PROGRAM P_Prog3
VAR

	fbKL6401 					: FB_LON_KL6401;

	fbREAD_063		: FB_READ_063_SNVT_temp_f;
	fbSEND_063		: FB_SEND_063_SNVT_temp_f;

	fbREAD_064		: FB_READ_064_SNVT_time_f;
	fbSEND_064		: FB_SEND_064_SNVT_time_f;

	fbREAD_065		: FB_READ_065_SNVT_vol_f;
	fbSEND_065		: FB_SEND_065_SNVT_vol_f;

	fbREAD_066		: FB_READ_066_SNVT_volt_f;
	fbSEND_066		: FB_SEND_066_SNVT_volt_f;

	fbREAD_067		: FB_READ_067_SNVT_btu_f;
	fbSEND_067		: FB_SEND_067_SNVT_btu_f;

	fbREAD_068		: FB_READ_068_SNVT_elec_whr_f;
	fbSEND_068		: FB_SEND_068_SNVT_elec_whr_f;

	fbREAD_069		: FB_READ_069_SNVT_config_src;
	fbSEND_069		: FB_SEND_069_SNVT_config_src;

	fbREAD_070		: FB_READ_070_SNVT_color;
	fbSEND_070		: FB_SEND_070_SNVT_color;

	fbREAD_071		: FB_READ_071_SNVT_grammage;
	fbSEND_071		: FB_SEND_071_SNVT_grammage;

	fbREAD_072		: FB_READ_072_SNVT_grammage_f;
	fbSEND_072		: FB_SEND_072_SNVT_grammage_f;

	fbREAD_073		: FB_READ_073_SNVT_file_req;
	fbSEND_073		: FB_SEND_073_SNVT_file_req;

	fbREAD_074		: FB_READ_074_SNVT_file_status;
	fbSEND_074		: FB_SEND_074_SNVT_file_status;

	fbREAD_075		: FB_READ_075_SNVT_freq_f;
	fbSEND_075		: FB_SEND_075_SNVT_freq_f;

	fbREAD_076		: FB_READ_076_SNVT_freq_hz;
	fbSEND_076		: FB_SEND_076_SNVT_freq_hz;

	fbREAD_077		: FB_READ_077_SNVT_freq_kilohz;
	fbSEND_077		: FB_SEND_077_SNVT_freq_kilohz;

	fbREAD_078		: FB_READ_078_SNVT_freq_milhz;
	fbSEND_078		: FB_SEND_078_SNVT_freq_milhz;

	fbREAD_079		: FB_READ_079_SNVT_lux;
	fbSEND_079		: FB_SEND_079_SNVT_lux;
(*
	fbREAD_080		: FB_READ_080;
	fbSEND_080		: FB_SEND_080_SNVT_angle_vel_f;
*)
	fbREAD_081		: FB_READ_081_SNVT_lev_percent;
	fbSEND_081		: FB_SEND_081_SNVT_lev_percent;

	fbREAD_082		: FB_READ_082_SNVT_multiplier;
	fbSEND_082		: FB_SEND_082_SNVT_multiplier;

	fbREAD_083		: FB_READ_083_SNVT_state;
	fbSEND_083		: FB_SEND_083_SNVT_state;

	fbREAD_084		: FB_READ_084_SNVT_time_stamp;
	fbSEND_084		: FB_SEND_084_SNVT_time_stamp;

	fbREAD_085		: FB_READ_085_SNVT_zerospan;
	fbSEND_085		: FB_SEND_085_SNVT_zerospan;

	fbREAD_086		: FB_READ_086_SNVT_magcard;
	fbSEND_086		: FB_SEND_086_SNVT_magcard;

	fbREAD_087		: FB_READ_087_SNVT_elapsed_tm;
	fbSEND_087		: FB_SEND_087_SNVT_elapsed_tm;

	fbREAD_088		: FB_READ_088_SNVT_alarm;
	fbSEND_088		: FB_SEND_088_SNVT_alarm;

	fbREAD_089		: FB_READ_089_SNVT_currency;
	fbSEND_089		: FB_SEND_089_SNVT_currency;

	fbREAD_090		: FB_READ_090_SNVT_file_pos;
	fbSEND_090		: FB_SEND_090_SNVT_file_pos;

	fbREAD_091		: FB_READ_091_SNVT_muldiv;
	fbSEND_091		: FB_SEND_091_SNVT_muldiv;

	fbREAD_092		: FB_READ_092_SNVT_obj_request;
	fbSEND_092		: FB_SEND_092_SNVT_obj_request;

	fbREAD_093		: FB_READ_093_SNVT_obj_status;
	fbSEND_093		: FB_SEND_093_SNVT_obj_status;

END_VAR

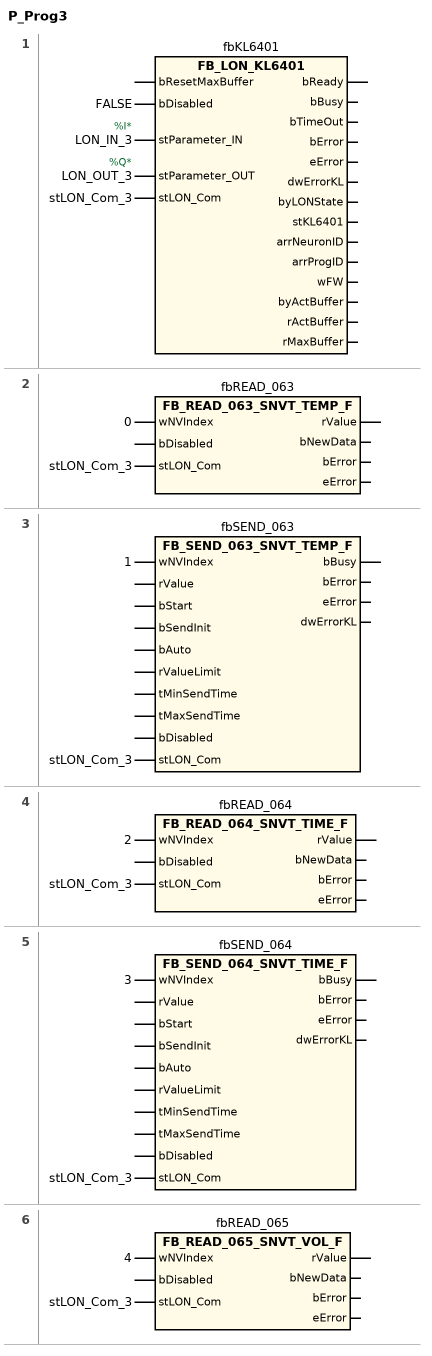
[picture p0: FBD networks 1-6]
// NETWORK 1
//   LON_IN_3: AT %I*
//   LON_OUT_3: AT %Q*
fbKL6401(
    bDisabled := FALSE,
    stParameter_IN := LON_IN_3,
    stParameter_OUT := LON_OUT_3,
    stLON_Com := stLON_Com_3); // FB_LON_KL6401

// NETWORK 2
fbREAD_063(wNVIndex := 0, stLON_Com := stLON_Com_3); // FB_READ_063_SNVT_TEMP_F

// NETWORK 3
fbSEND_063(wNVIndex := 1, stLON_Com := stLON_Com_3); // FB_SEND_063_SNVT_TEMP_F

// NETWORK 4
fbREAD_064(wNVIndex := 2, stLON_Com := stLON_Com_3); // FB_READ_064_SNVT_TIME_F

// NETWORK 5
fbSEND_064(wNVIndex := 3, stLON_Com := stLON_Com_3); // FB_SEND_064_SNVT_TIME_F

// NETWORK 6
fbREAD_065(wNVIndex := 4, stLON_Com := stLON_Com_3); // FB_READ_065_SNVT_VOL_F

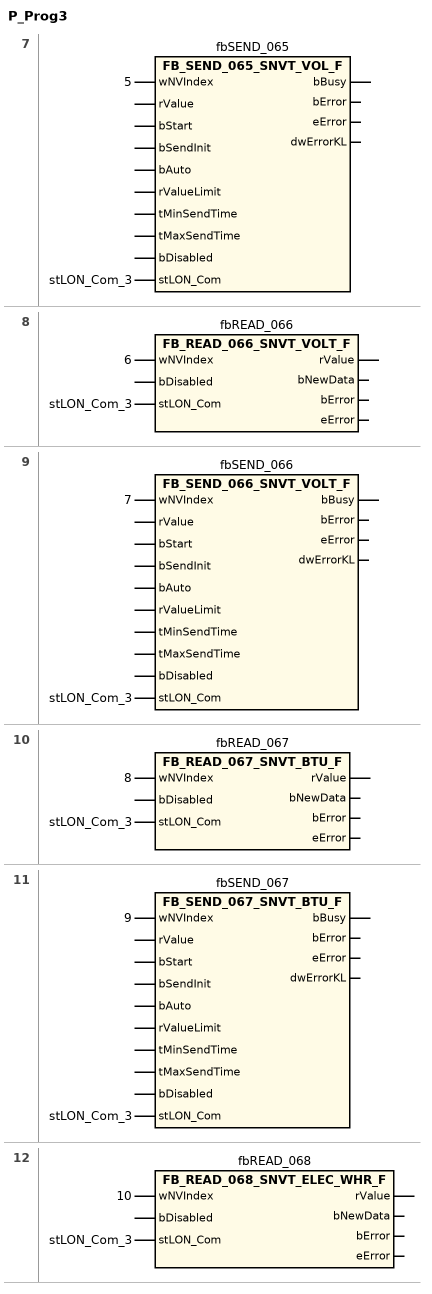
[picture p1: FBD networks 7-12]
// NETWORK 7
fbSEND_065(wNVIndex := 5, stLON_Com := stLON_Com_3); // FB_SEND_065_SNVT_VOL_F

// NETWORK 8
fbREAD_066(wNVIndex := 6, stLON_Com := stLON_Com_3); // FB_READ_066_SNVT_VOLT_F

// NETWORK 9
fbSEND_066(wNVIndex := 7, stLON_Com := stLON_Com_3); // FB_SEND_066_SNVT_VOLT_F

// NETWORK 10
fbREAD_067(wNVIndex := 8, stLON_Com := stLON_Com_3); // FB_READ_067_SNVT_BTU_F

// NETWORK 11
fbSEND_067(wNVIndex := 9, stLON_Com := stLON_Com_3); // FB_SEND_067_SNVT_BTU_F

// NETWORK 12
fbREAD_068(wNVIndex := 10, stLON_Com := stLON_Com_3); // FB_READ_068_SNVT_ELEC_WHR_F

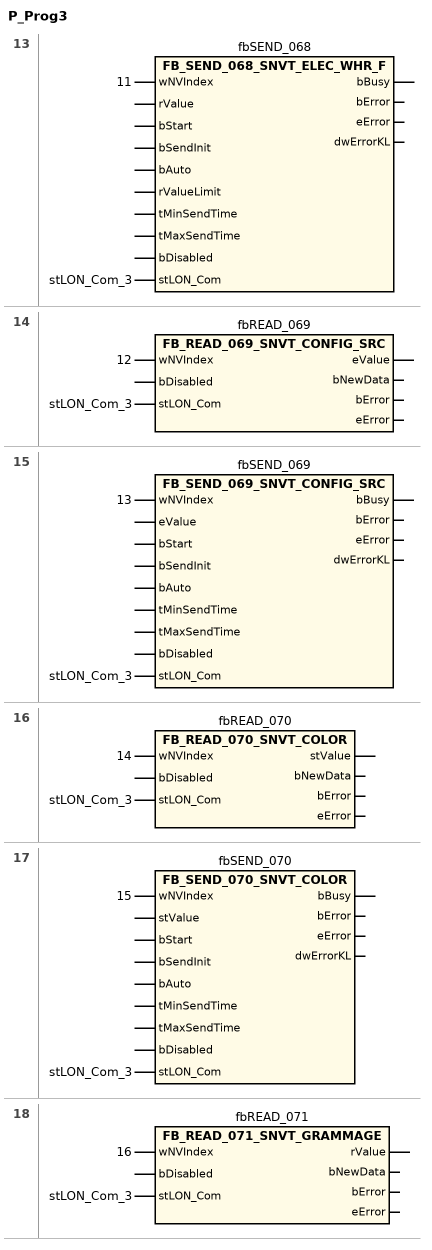
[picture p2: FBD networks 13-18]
// NETWORK 13
fbSEND_068(wNVIndex := 11, stLON_Com := stLON_Com_3); // FB_SEND_068_SNVT_ELEC_WHR_F

// NETWORK 14
fbREAD_069(wNVIndex := 12, stLON_Com := stLON_Com_3); // FB_READ_069_SNVT_CONFIG_SRC

// NETWORK 15
fbSEND_069(wNVIndex := 13, stLON_Com := stLON_Com_3); // FB_SEND_069_SNVT_CONFIG_SRC

// NETWORK 16
fbREAD_070(wNVIndex := 14, stLON_Com := stLON_Com_3); // FB_READ_070_SNVT_COLOR

// NETWORK 17
fbSEND_070(wNVIndex := 15, stLON_Com := stLON_Com_3); // FB_SEND_070_SNVT_COLOR

// NETWORK 18
fbREAD_071(wNVIndex := 16, stLON_Com := stLON_Com_3); // FB_READ_071_SNVT_GRAMMAGE

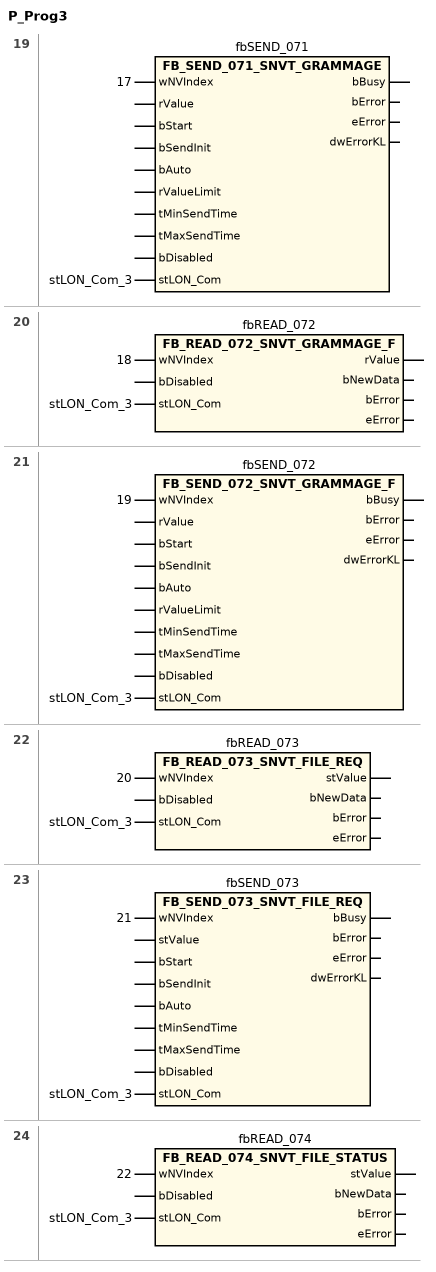
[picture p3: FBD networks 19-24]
// NETWORK 19
fbSEND_071(wNVIndex := 17, stLON_Com := stLON_Com_3); // FB_SEND_071_SNVT_GRAMMAGE

// NETWORK 20
fbREAD_072(wNVIndex := 18, stLON_Com := stLON_Com_3); // FB_READ_072_SNVT_GRAMMAGE_F

// NETWORK 21
fbSEND_072(wNVIndex := 19, stLON_Com := stLON_Com_3); // FB_SEND_072_SNVT_GRAMMAGE_F

// NETWORK 22
fbREAD_073(wNVIndex := 20, stLON_Com := stLON_Com_3); // FB_READ_073_SNVT_FILE_REQ

// NETWORK 23
fbSEND_073(wNVIndex := 21, stLON_Com := stLON_Com_3); // FB_SEND_073_SNVT_FILE_REQ

// NETWORK 24
fbREAD_074(wNVIndex := 22, stLON_Com := stLON_Com_3); // FB_READ_074_SNVT_FILE_STATUS

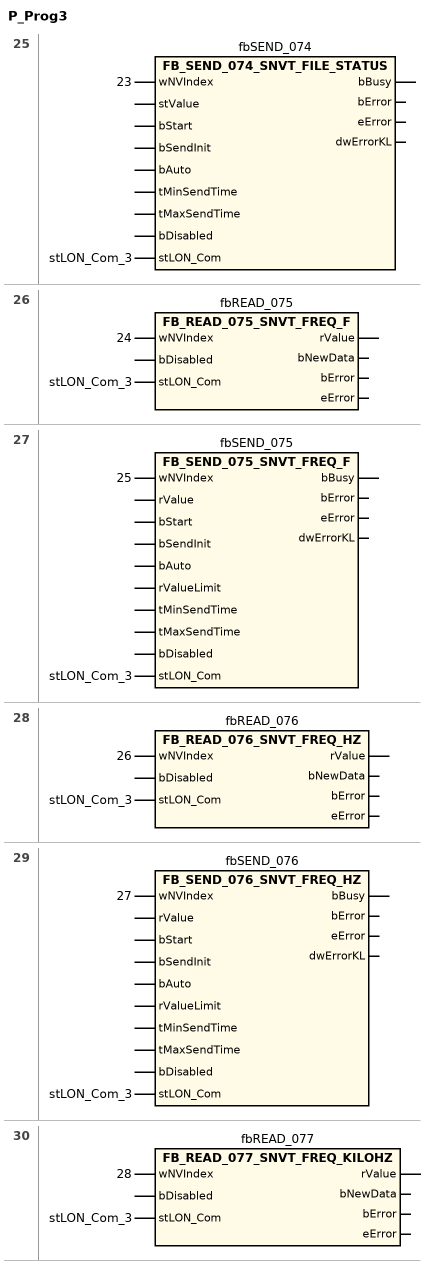
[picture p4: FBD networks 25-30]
// NETWORK 25
fbSEND_074(wNVIndex := 23, stLON_Com := stLON_Com_3); // FB_SEND_074_SNVT_FILE_STATUS

// NETWORK 26
fbREAD_075(wNVIndex := 24, stLON_Com := stLON_Com_3); // FB_READ_075_SNVT_FREQ_F

// NETWORK 27
fbSEND_075(wNVIndex := 25, stLON_Com := stLON_Com_3); // FB_SEND_075_SNVT_FREQ_F

// NETWORK 28
fbREAD_076(wNVIndex := 26, stLON_Com := stLON_Com_3); // FB_READ_076_SNVT_FREQ_HZ

// NETWORK 29
fbSEND_076(wNVIndex := 27, stLON_Com := stLON_Com_3); // FB_SEND_076_SNVT_FREQ_HZ

// NETWORK 30
fbREAD_077(wNVIndex := 28, stLON_Com := stLON_Com_3); // FB_READ_077_SNVT_FREQ_KILOHZ

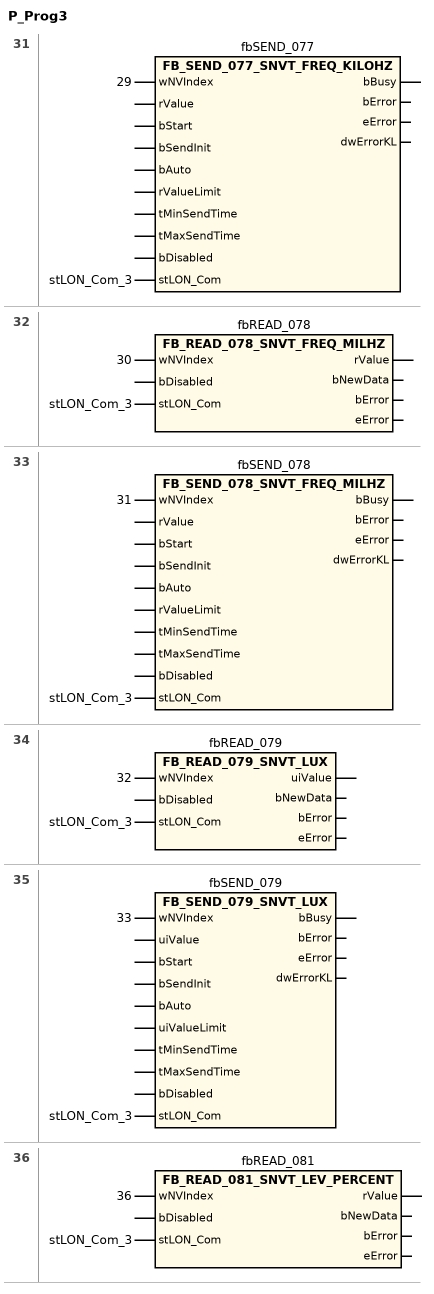
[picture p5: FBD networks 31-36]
// NETWORK 31
fbSEND_077(wNVIndex := 29, stLON_Com := stLON_Com_3); // FB_SEND_077_SNVT_FREQ_KILOHZ

// NETWORK 32
fbREAD_078(wNVIndex := 30, stLON_Com := stLON_Com_3); // FB_READ_078_SNVT_FREQ_MILHZ

// NETWORK 33
fbSEND_078(wNVIndex := 31, stLON_Com := stLON_Com_3); // FB_SEND_078_SNVT_FREQ_MILHZ

// NETWORK 34
fbREAD_079(wNVIndex := 32, stLON_Com := stLON_Com_3); // FB_READ_079_SNVT_LUX

// NETWORK 35
fbSEND_079(wNVIndex := 33, stLON_Com := stLON_Com_3); // FB_SEND_079_SNVT_LUX

// NETWORK 36
//   fbREAD_081: fbREAD_080 : FB_READ_080; fbSEND_080 : FB_SEND_080_SNVT_angle_vel_f;
fbREAD_081(wNVIndex := 36, stLON_Com := stLON_Com_3); // FB_READ_081_SNVT_LEV_PERCENT

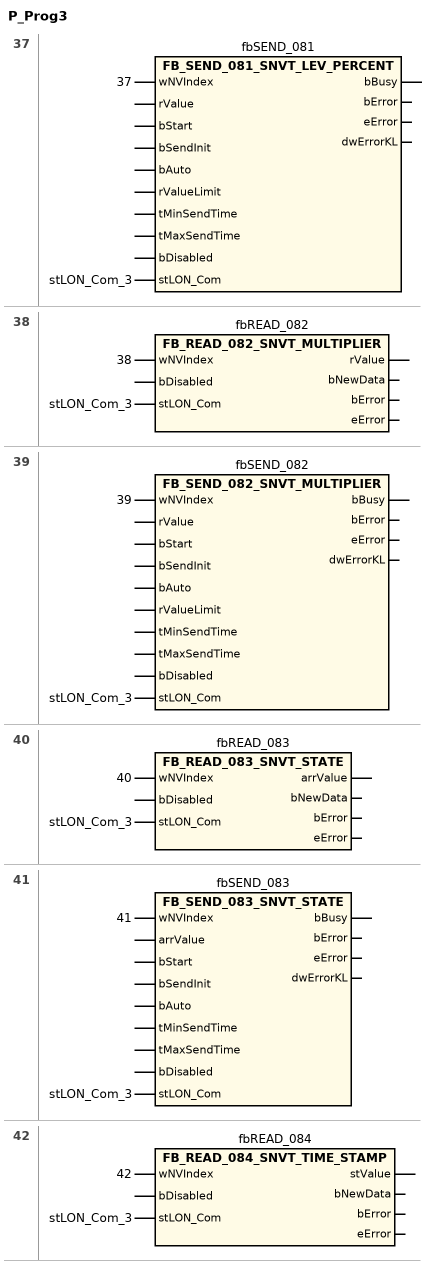
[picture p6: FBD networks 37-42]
// NETWORK 37
fbSEND_081(wNVIndex := 37, stLON_Com := stLON_Com_3); // FB_SEND_081_SNVT_LEV_PERCENT

// NETWORK 38
fbREAD_082(wNVIndex := 38, stLON_Com := stLON_Com_3); // FB_READ_082_SNVT_MULTIPLIER

// NETWORK 39
fbSEND_082(wNVIndex := 39, stLON_Com := stLON_Com_3); // FB_SEND_082_SNVT_MULTIPLIER

// NETWORK 40
fbREAD_083(wNVIndex := 40, stLON_Com := stLON_Com_3); // FB_READ_083_SNVT_STATE

// NETWORK 41
fbSEND_083(wNVIndex := 41, stLON_Com := stLON_Com_3); // FB_SEND_083_SNVT_STATE

// NETWORK 42
fbREAD_084(wNVIndex := 42, stLON_Com := stLON_Com_3); // FB_READ_084_SNVT_TIME_STAMP

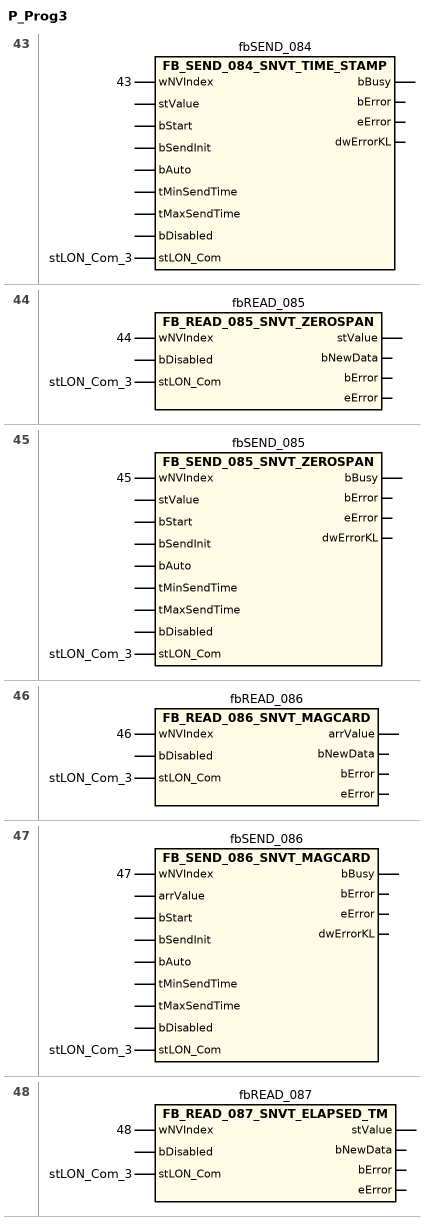
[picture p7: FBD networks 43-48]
// NETWORK 43
fbSEND_084(wNVIndex := 43, stLON_Com := stLON_Com_3); // FB_SEND_084_SNVT_TIME_STAMP

// NETWORK 44
fbREAD_085(wNVIndex := 44, stLON_Com := stLON_Com_3); // FB_READ_085_SNVT_ZEROSPAN

// NETWORK 45
fbSEND_085(wNVIndex := 45, stLON_Com := stLON_Com_3); // FB_SEND_085_SNVT_ZEROSPAN

// NETWORK 46
fbREAD_086(wNVIndex := 46, stLON_Com := stLON_Com_3); // FB_READ_086_SNVT_MAGCARD

// NETWORK 47
fbSEND_086(wNVIndex := 47, stLON_Com := stLON_Com_3); // FB_SEND_086_SNVT_MAGCARD

// NETWORK 48
fbREAD_087(wNVIndex := 48, stLON_Com := stLON_Com_3); // FB_READ_087_SNVT_ELAPSED_TM

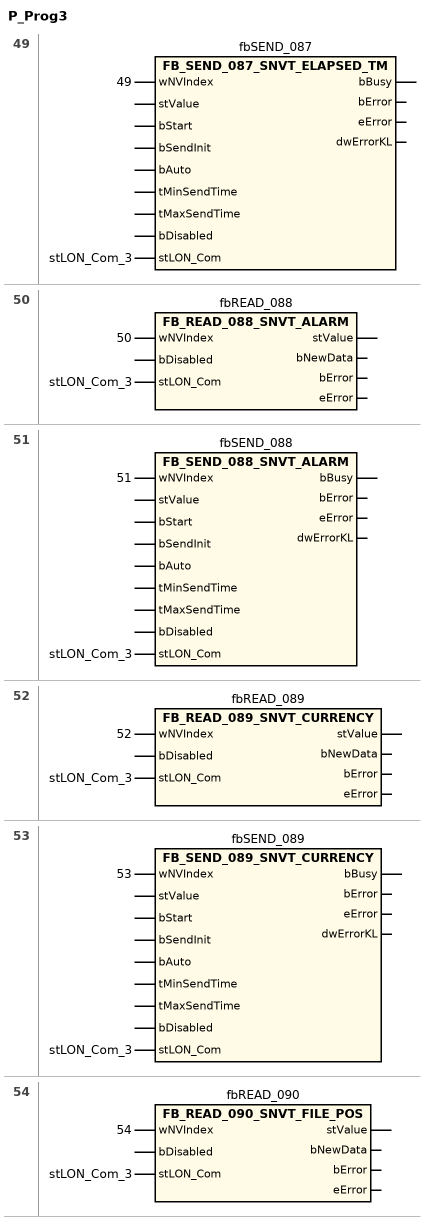
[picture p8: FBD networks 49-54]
// NETWORK 49
fbSEND_087(wNVIndex := 49, stLON_Com := stLON_Com_3); // FB_SEND_087_SNVT_ELAPSED_TM

// NETWORK 50
fbREAD_088(wNVIndex := 50, stLON_Com := stLON_Com_3); // FB_READ_088_SNVT_ALARM

// NETWORK 51
fbSEND_088(wNVIndex := 51, stLON_Com := stLON_Com_3); // FB_SEND_088_SNVT_ALARM

// NETWORK 52
fbREAD_089(wNVIndex := 52, stLON_Com := stLON_Com_3); // FB_READ_089_SNVT_CURRENCY

// NETWORK 53
fbSEND_089(wNVIndex := 53, stLON_Com := stLON_Com_3); // FB_SEND_089_SNVT_CURRENCY

// NETWORK 54
fbREAD_090(wNVIndex := 54, stLON_Com := stLON_Com_3); // FB_READ_090_SNVT_FILE_POS

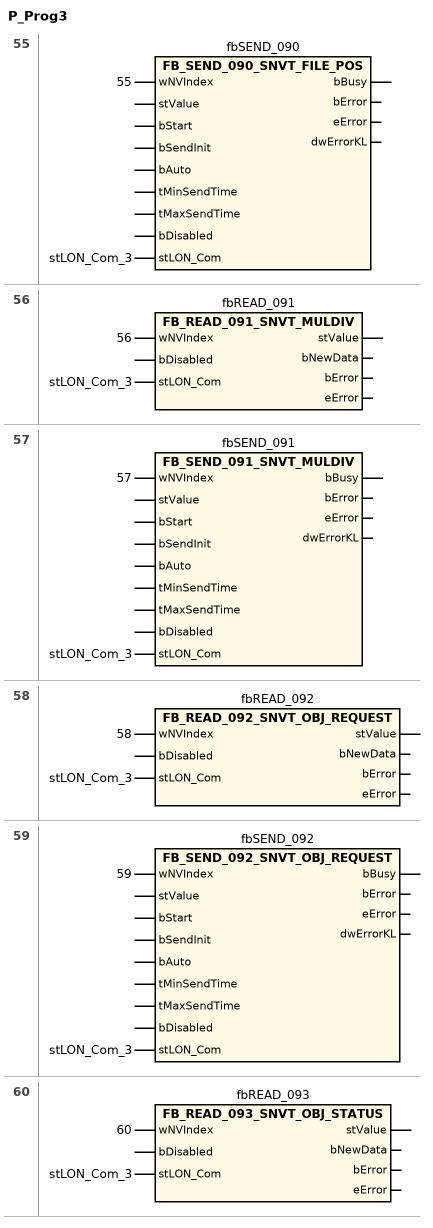
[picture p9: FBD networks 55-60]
// NETWORK 55
fbSEND_090(wNVIndex := 55, stLON_Com := stLON_Com_3); // FB_SEND_090_SNVT_FILE_POS

// NETWORK 56
fbREAD_091(wNVIndex := 56, stLON_Com := stLON_Com_3); // FB_READ_091_SNVT_MULDIV

// NETWORK 57
fbSEND_091(wNVIndex := 57, stLON_Com := stLON_Com_3); // FB_SEND_091_SNVT_MULDIV

// NETWORK 58
fbREAD_092(wNVIndex := 58, stLON_Com := stLON_Com_3); // FB_READ_092_SNVT_OBJ_REQUEST

// NETWORK 59
fbSEND_092(wNVIndex := 59, stLON_Com := stLON_Com_3); // FB_SEND_092_SNVT_OBJ_REQUEST

// NETWORK 60
fbREAD_093(wNVIndex := 60, stLON_Com := stLON_Com_3); // FB_READ_093_SNVT_OBJ_STATUS

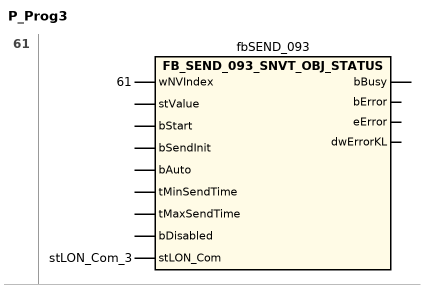
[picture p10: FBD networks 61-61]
// NETWORK 61
fbSEND_093(wNVIndex := 61, stLON_Com := stLON_Com_3); // FB_SEND_093_SNVT_OBJ_STATUS

END_PROGRAM
